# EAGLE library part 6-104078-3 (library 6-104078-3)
Check availability
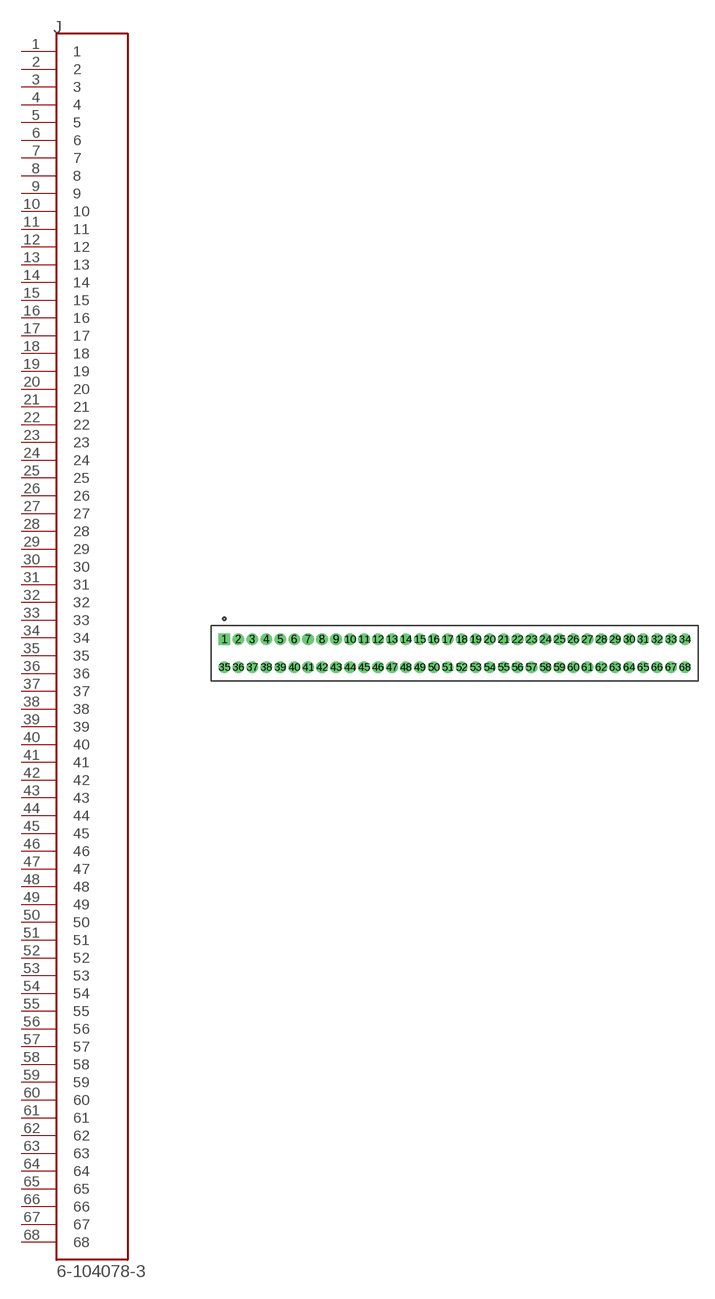
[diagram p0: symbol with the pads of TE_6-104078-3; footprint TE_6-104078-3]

Designator prefix J

## 6-104078-3 (Availability: In Stock; Comment: 6-104078-3; Description: Conn Socket Strip RCP 68 POS 1.27mm Solder ST Thru-Hole Tube; EU_RoHS_Compliance: Compliant; MF: TE Connectivity; MP: 6-104078-3; Package: None; Price: None; Purchase-URL: https://pricing.snapeda.com/search/part/6-104078-3/?ref=eda)  [TE_6-104078-3]
1  1  pas
2  2  pas
3  3  pas
4  4  pas
5  5  pas
6  6  pas
7  7  pas
8  8  pas
9  9  pas
10  10  pas
11  11  pas
12  12  pas
13  13  pas
14  14  pas
15  15  pas
16  16  pas
17  17  pas
18  18  pas
19  19  pas
20  20  pas
21  21  pas
22  22  pas
23  23  pas
24  24  pas
25  25  pas
26  26  pas
27  27  pas
28  28  pas
29  29  pas
30  30  pas
31  31  pas
32  32  pas
33  33  pas
34  34  pas
35  35  pas
36  36  pas
37  37  pas
38  38  pas
39  39  pas
40  40  pas
41  41  pas
42  42  pas
43  43  pas
44  44  pas
45  45  pas
46  46  pas
47  47  pas
48  48  pas
49  49  pas
50  50  pas
51  51  pas
52  52  pas
53  53  pas
54  54  pas
55  55  pas
56  56  pas
57  57  pas
58  58  pas
59  59  pas
60  60  pas
61  61  pas
62  62  pas
63  63  pas
64  64  pas
65  65  pas
66  66  pas
67  67  pas
68  68  pas

## Footprint TE_6-104078-3 (pad centres in mm)
drill 0.56 pad 0.89 square: 1 -20.955,1.27
drill 0.56 pad 0.89: 2 -19.685,1.27; 3 -18.415,1.27; 4 -17.145,1.27; 5 -15.875,1.27; 6 -14.605,1.27; 7 -13.335,1.27; 8 -12.065,1.27; 9 -10.795,1.27; 10 -9.525,1.27; 11 -8.255,1.27; 12 -6.985,1.27; 13 -5.715,1.27; 14 -4.445,1.27; 15 -3.175,1.27; 16 -1.905,1.27; 17 -0.635,1.27; 18 0.635,1.27; 19 1.905,1.27; 20 3.175,1.27; 21 4.445,1.27; 22 5.715,1.27; 23 6.985,1.27; 24 8.255,1.27; 25 9.525,1.27; 26 10.795,1.27; 27 12.065,1.27; 28 13.335,1.27; 29 14.605,1.27; 30 15.875,1.27; 31 17.145,1.27; 32 18.415,1.27; 33 19.685,1.27; 34 20.955,1.27; 35 -20.955,-1.27; 36 -19.685,-1.27; 37 -18.415,-1.27; 38 -17.145,-1.27; 39 -15.875,-1.27; 40 -14.605,-1.27; 41 -13.335,-1.27; 42 -12.065,-1.27; 43 -10.795,-1.27; 44 -9.525,-1.27; 45 -8.255,-1.27; 46 -6.985,-1.27; 47 -5.715,-1.27; 48 -4.445,-1.27; 49 -3.175,-1.27; 50 -1.905,-1.27; 51 -0.635,-1.27; 52 0.635,-1.27; 53 1.905,-1.27; 54 3.175,-1.27; 55 4.445,-1.27; 56 5.715,-1.27; 57 6.985,-1.27; 58 8.255,-1.27; 59 9.525,-1.27; 60 10.795,-1.27; 61 12.065,-1.27; 62 13.335,-1.27; 63 14.605,-1.27; 64 15.875,-1.27; 65 17.145,-1.27; 66 18.415,-1.27; 67 19.685,-1.27; 68 20.955,-1.27

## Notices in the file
This work is licensed under a Creative Commons Attribution-ShareAlike 4.0 International License (CC BY-SA) with Design Exception 1.0
